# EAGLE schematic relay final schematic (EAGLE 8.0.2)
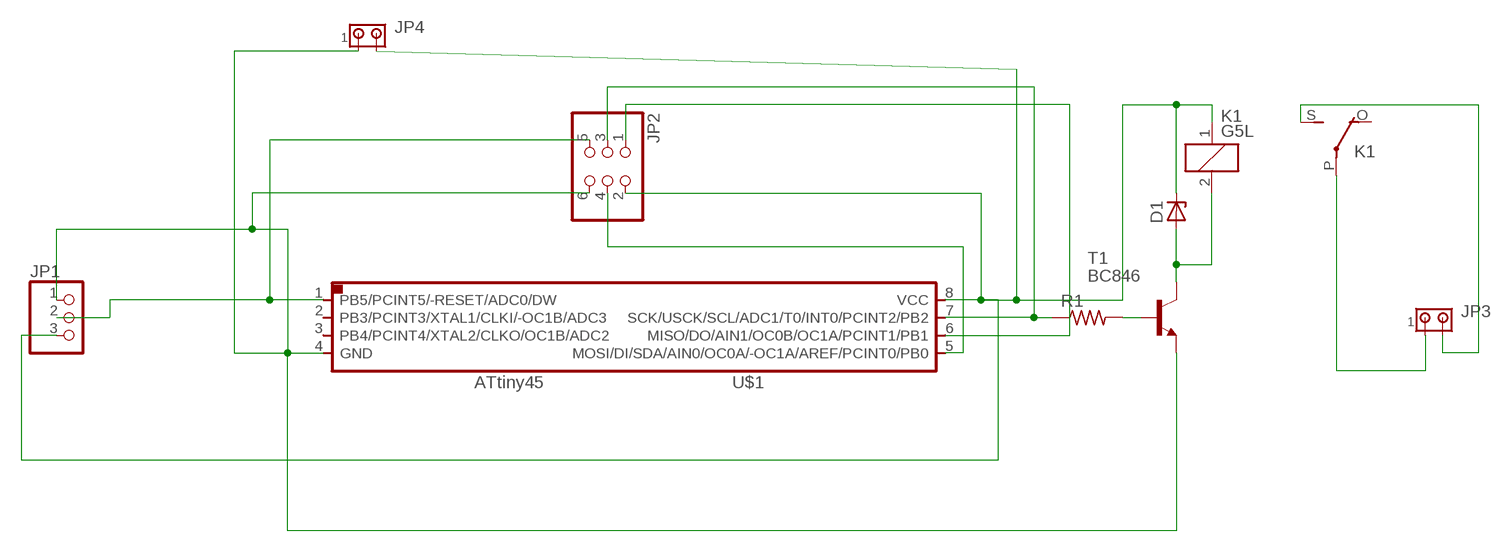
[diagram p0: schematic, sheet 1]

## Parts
D1  ZENER_DIODESOD123  [SOD123]
JP1  PINHD-1X3  [1X03]
JP2  PINHD-2X3-SMD  [2X03SMD]
JP3  MTA02-156  [1X2MTA]
JP4  MTA02-156  [1X2MTA]
K1  G5L  [G5LE]
R1  RES-US1206  [R1206]
T1  BC846  [SOT23]
U$1  ATTINY45SI  [SOIC8]

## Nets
N$1: JP1.1 JP2.6 JP4.1 T1.2(E) U$1.4(GND)
N$2: D1.CATHODE JP1.3 JP2.2 JP4.2 K1.1 U$1.8(VCC)
N$3: JP1.2 JP2.5 U$1.1(PB5/PCINT5/-RESET/ADC0/DW)
N$4: JP2.4 U$1.5(MOSI/DI/SDA/AIN0/OC0A/-OC1A/AREF/PCINT0/PB0)
N$5: JP2.3 R1.1 U$1.7(SCK/USCK/SCL/ADC1/T0/INT0/PCINT2/PB2)
N$6: JP2.1 U$1.6(MISO/DO/AIN1/OC0B/OC1A/PCINT1/PB1)
N$7: JP3.1 K1.P(2:P)
N$9: D1.ANODE K1.2 T1.3(C)
N$10: R1.2 T1.1(B)
N$11: JP3.2 K1.S(2:S)
Unconnected: K1.O(2:O) U$1.2(PB3/PCINT3/XTAL1/CLKI/-OC1B/ADC3) U$1.3(PB4/PCINT4/XTAL2/CLKO/OC1B/ADC2)

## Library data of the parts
D1 = fab:ZENER_DIODE: zener diode
JP1 = pinhead:PINHD-1X3: PIN HEADER
JP2 = fab:PINHD-2X3-SMD: PIN HEADER
JP3 JP4 = con-amp:MTA02-156: AMP connector
K1 = relay:G5L: RELAY 1 x switch, 10 A/120 V AC, 8 A/30 V ADC, Omron; OC_FARNELL: unknown; OC_NEWARK: unknown
R1 = fab:RES-US: Resistor (US Symbol)
T1 = transistor:BC846: NPN TRANSISTOR
U$1 = fab:ATTINY45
